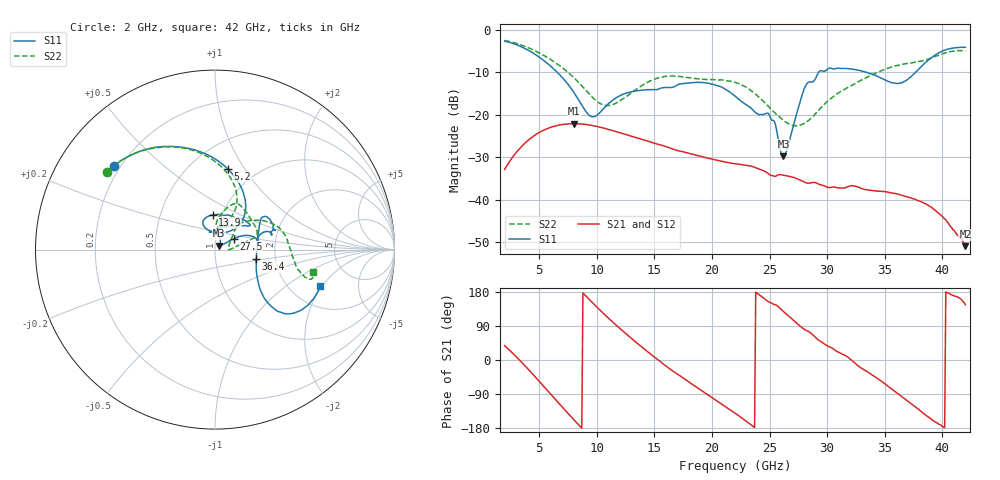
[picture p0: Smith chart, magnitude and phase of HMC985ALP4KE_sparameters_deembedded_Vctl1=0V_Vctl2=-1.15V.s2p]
!s2p File: Measurements: S11, S21, S12, S22
# GHz S dB R 50.0
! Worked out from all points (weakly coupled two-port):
!   401 points, 2 GHz to 42 GHz, reference 50 ohm
!   highest |S21| = -22.11 dB at 8 GHz (marker M1); lowest = -50.9 dB at 42 GHz (marker M2)
!   lowest |S11| = -29.8 dB at 26.2 GHz (marker M3), VSWR 1.07, Z = 52.4 + j2.28 ohm
!   |S11| at or under -10 dB: 6.554 GHz to 29.27 GHz (22.72 GHz wide, 127 % of centre); 33.35 GHz to 37.69 GHz (4.345 GHz wide, 12.2 % of centre)
!   |S22| runs from -22.7 to -2.6 dB; largest |S21 - S12| = 0.00015
!   S11 on the Smith chart (normalised r, x): 2 GHz: 0.17, +0.35; 5.2 GHz: 0.75, +0.85; 13.9 GHz: 0.90, +0.36; 27.5 GHz: 1.22, +0.15; 36.4 GHz: 1.58, -0.18; 42 GHz: 2.90, -1.91
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2  -2.71 140.4  -32.89 37.8  -32.88 37.8  -2.56 144.3
3.5  -4.11 112.6  -27.39 -6.6  -27.40 -6.6  -3.70 119.6
5.2  -6.87 80.7  -23.89 -62.9  -23.90 -62.9  -5.78 93.6
8  -14.71 45.8  -22.11 -157.3  -22.11 -157.3  -11.26 64.2
8.7  -17.77 51.8  -22.19 -179.8  -22.20 -179.8  -13.21 62.9
9.7  -20.51 85.4  -22.58 149.0  -22.58 149.0  -16.11 68.3
10.9  -17.70 113.6  -23.37 113.6  -23.37 113.6  -17.86 82.2
13.9  -14.25 93.9  -25.77 34.5  -25.78 34.5  -13.18 77.4
15.4  -13.94 73.0  -27.00 -1.4  -27.00 -1.4  -11.30 68.4
19.4  -12.52 34.6  -30.05 -87.0  -30.06 -87.0  -11.70 36.5
22  -15.61 52.3  -31.50 -140.0  -31.51 -140.1  -12.41 18.2
25  -20.18 97.9  -34.11 152.0  -34.11 152.0  -18.34 8.6
26.2  -29.80 42.1  -34.20 128.0  -34.21 128.0  -21.33 1.3
27.5  -18.39 29.8  -35.15 93.3  -35.18 93.3  -22.55 6.0
28.1  -13.35 20.8  -35.93 79.3  -35.93 79.3  -21.92 15.7
28.7  -12.31 12.9  -35.95 68.1  -35.95 68.1  -20.56 25.8
31  -9.08 23.3  -37.22 20.5  -37.19 20.3  -14.84 46.3
33.3  -9.96 34.4  -37.59 -27.4  -37.57 -27.5  -11.45 37.3
35.4  -12.27 12.3  -38.28 -71.7  -38.27 -71.7  -9.01 23.5
36.4  -12.57 -12.8  -38.88 -94.5  -38.87 -94.5  -8.23 15.8
39.5  -5.81 -43.3  -42.79 -165.6  -42.75 -165.4  -6.20 -14.5
42  -4.14 -19.0  -50.88 145.8  -51.04 146.0  -5.02 -13.1
